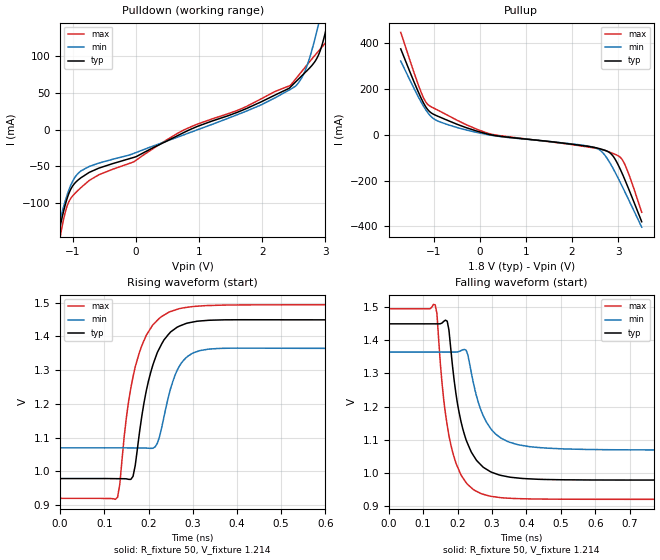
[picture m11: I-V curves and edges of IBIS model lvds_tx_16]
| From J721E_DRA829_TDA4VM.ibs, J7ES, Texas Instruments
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|   MODEL lvds_tx_16
[Model] lvds_tx_16
Model_type Output
C_comp 1.683p 1.757p 1.495p
Vmeas = 1.2
Vref = 1.2V
Rref = 50
Cref = 0.5pF
[Model Spec]
[Temperature Range]  40 150 -40
[Voltage Range] 1.8 1.62 1.98
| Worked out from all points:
|   slope of the pulldown table from 0 to 0.27 V, typ, clamps not added: 22.2 ohm
|   slope of the pullup table from 0 to 0.27 V, typ, clamps not added: 19.7 ohm
|   rising waveform, R_fixture 50, V_fixture 1.214: 20-80 % time 45.7ps typ, 37.6ps min, 47.1ps max; typ from 0.979 V to 1.45 V
|   falling waveform, R_fixture 50, V_fixture 1.214: 20-80 % time 53.4ps typ, 60.6ps min, 46.9ps max; typ from 1.45 V to 0.979 V
[Pulldown]
-1.71V    -379.4mA   -326.9mA   -450.3mA
-1.245V   -150.8mA   -138.5mA   -169.7mA
-1.193V   -128.7mA   -120.1mA   -142.8mA
-1.05V    -84.41mA   -79.45mA   -96.13mA
-870.6mV  -65.45mA   -56.1mA    -78.87mA
769mV     -3.402mA   -6.65mA    0A
2.202V    47.14mA    43.31mA    52.01mA
2.624V    73.08mA    70.22mA    78.99mA
2.888V    100.8mA    141.6mA    106.6mA
3.03V     143.3mA    196.1mA    121.1mA
3.141V    190.9mA    241.2mA    140.2mA
3.511V    373.6mA    396.2mA    335.4mA
[Pullup]
-1.711V   373.6mA    320.5mA    445.6mA
-1.283V   165mA      147.2mA    191.6mA
-1.183V   125.9mA    112.8mA    147mA
-1.098V   102.9mA    88.87mA    127.1mA
-670.8mV  60.05mA    42.1mA     81.86mA
224.4mV   0A         -1.895mA   3.363mA
2.565V    -59.44mA   -62.41mA   -61.27mA
2.702V    -67.66mA   -87.1mA    -68.11mA
2.861V    -86.69mA   -136.8mA   -79.83mA
3.088V    -169.7mA   -225.4mA   -109mA
3.225V    -235.3mA   -282.6mA   -169.4mA
3.51V     -379.4mA   -403mA     -338.4mA
[Ramp]
dV/dt_r .283/45.809p .177/37.495p .345/47.322p
dV/dt_f .283/53.387p .177/60.54p .345/46.898p
[Rising Waveform]
R_fixture = 50
V_fixture = 1.214
V_fixture_min = 1.217
V_fixture_max = 1.208
0s        978.9mV    1.07V      920.2mV
130ps     978.5mV    1.07V      923.6mV
160ps     976.4mV    1.07V      1.247V
170ps     1.018V     1.07V      1.31V
180ps     1.12V      1.069V     1.355V
210ps     1.316V     1.069V     1.434V
235ps     1.39V      1.162V     1.463V
280ps     1.436V     1.33V      1.485V
385ps     1.449V     1.365V     1.493V
2.56ns    1.45V      1.364V     1.495V
[Falling Waveform]
R_fixture = 50
V_fixture = 1.214
V_fixture_min = 1.217
V_fixture_max = 1.208
0s        1.45V      1.365V     1.495V
135ps     1.45V      1.365V     1.508V
170ps     1.458V     1.365V     1.144V
185ps     1.326V     1.365V     1.065V
200ps     1.208V     1.365V     1.018V
225ps     1.099V     1.37V      970.2mV
260ps     1.032V     1.214V     941.6mV
295ps     1.004V     1.136V     929.4mV
510ps     979mV      1.072V     920.3mV
2.56ns    978.8mV    1.07V      920mV
